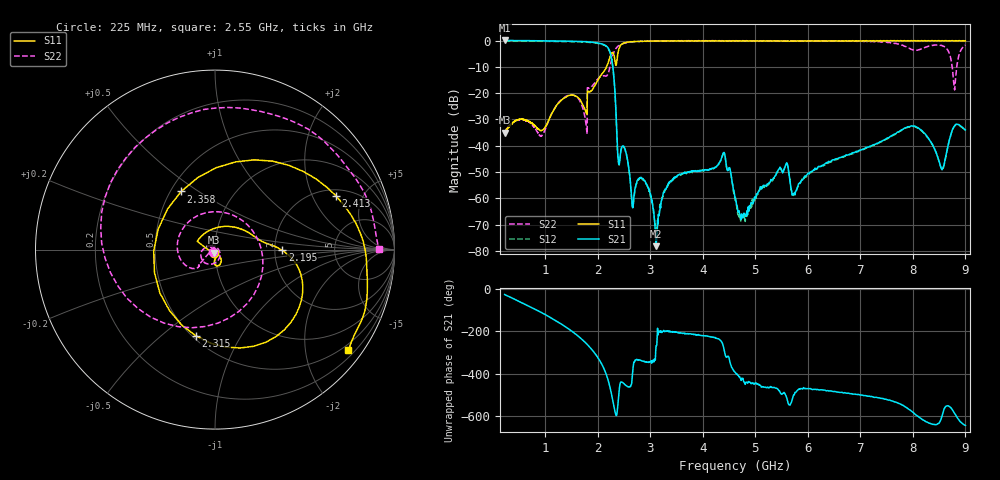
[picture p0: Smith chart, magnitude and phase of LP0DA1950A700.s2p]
!Agilent Technologies,E8358A,US41080443,A.07.50.56
!Agilent E8358A: A.07.50.56
!Date: Wednesday, May 04, 2016 15:05:05
!Correction: S11(Full 2 Port(1,2))
!S21(Full 2 Port(1,2))
!S12(Full 2 Port(1,2))
!S22(Full 2 Port(1,2))
!S2P File: Measurements: S11, S21, S12, S22:Log Frequency Sweep
# Hz S  dB  R 50
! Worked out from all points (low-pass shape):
!   1601 points, 225 MHz to 9 GHz, reference 50 ohm
!   highest |S21| = 0.03 dB at 229.2 MHz (marker M1); lowest = -78.2 dB at 3.109 GHz (marker M2)
!   |S21| within 3 dB of the highest: start of sweep to 2.2 GHz
!   lowest |S11| = -35.0 dB at 225 MHz (marker M3), VSWR 1.04, Z = 49.5 - j1.7 ohm
!   |S11| at or under -10 dB: start of sweep to 2.166 GHz
!   |S22| runs from -36.4 to 0.0 dB; largest |S21 - S12| = 0.019
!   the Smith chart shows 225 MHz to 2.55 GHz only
!   S11 on the Smith chart (normalised r, x): 225 MHz: 0.99, -0.03; 2.195 GHz: 2.20, -0.02; 2.315 GHz: 0.52, -0.66; 2.358 GHz: 0.57, +0.43; 2.413 GHz: 2.32, +3.05; 2.55 GHz: 0.36, -2.96
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2.25e8  -35.03 -104.9  0.02 -26.2  -0.13 -26.0  -34.78 -127.1
2.291885e8  -34.81 -105.2  0.03 -26.7  -0.13 -26.5  -34.64 -127.9
9.310556e8  -34.16 -92.6  -0.09 -111.9  -0.25 -111.7  -36.13 44.3
1.362034e9  -21.85 -67.0  -0.22 -174.6  -0.38 -174.5  -21.64 -102.8
1.687749e9  -23.36 -93.8  -0.37 124.5  -0.52 124.7  -24.19 174.6
2.043688e9  -13.64 27.6  -1.11 19.1  -1.27 19.3  -13.77 -170.9
2.195101e9  -8.53 -0.6  -2.80 -69.6  -2.95 -69.5  -12.62 27.9
2.314644e9  -6.17 -102.7  -16.05 156.0  -16.19 156.5  -3.98 176.8
2.357732e9  -8.52 120.2  -33.38 124.6  -33.54 124.6  -2.70 122.0
2.412722e9  -2.65 24.0  -46.45 -105.3  -46.62 -105.2  -1.82 71.5
2.549989e9  -0.64 -36.9  -43.73 -97.8  -43.92 -98.0  -0.80 0.3
3.109202e9  -0.27 -97.0  -78.16 91.2  -72.66 74.3  -0.21 -89.1
3.152512e9  -0.16 -99.8  -66.09 159.4  -67.52 156.5  -0.15 -92.5
3.409577e9  -0.12 -111.2  -53.13 157.1  -53.34 156.8  -0.11 -108.3
4.353484e9  -0.21 -136.0  -44.81 112.0  -44.85 110.7  -0.10 -145.2
4.622431e9  -0.16 -141.3  -59.91 -35.8  -60.92 -40.8  -0.06 -154.6
6.081681e9  -0.11 -174.3  -49.73 -114.4  -49.82 -113.8  -0.20 144.9
7.553438e9  -0.15 164.0  -36.75 -164.1  -36.84 -165.2  -0.74 59.6
8.057136e9  -0.15 159.5  -32.80 125.4  -32.89 125.7  -3.66 -83.6
8.302281e9  -0.06 158.1  -37.29 87.0  -37.42 87.4  -2.13 179.8
8.535184e9  -0.14 158.2  -48.35 104.8  -48.30 103.9  -1.81 127.8
9e9  -0.08 155.4  -34.00 75.8  -34.13 76.1  -1.74 159.8
